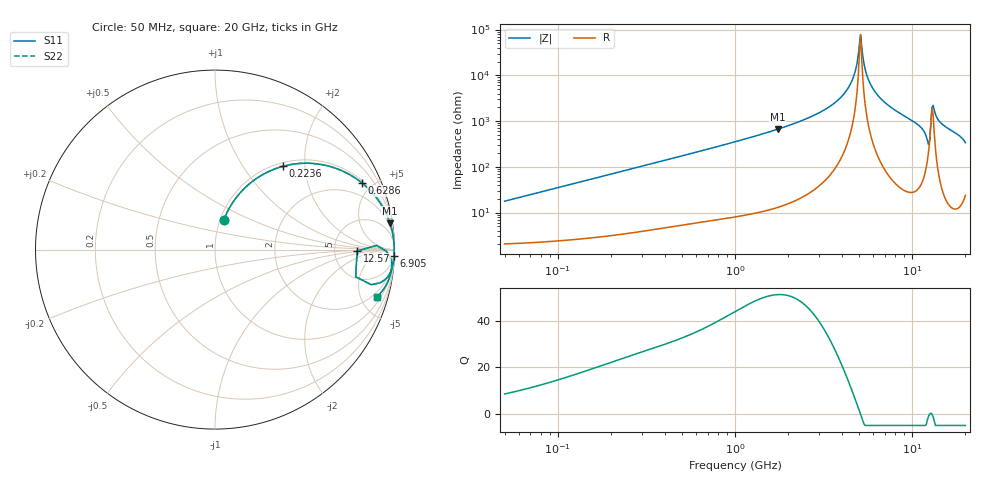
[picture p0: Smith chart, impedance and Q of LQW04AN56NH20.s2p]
!Murata Part Number: LQW04AN56NH20
!These Parameters are Measured in Series Mode Connection
!  o--[Z]--o
!Port1  Port2
!  o-------o
!Freq. Start=50[MHz] Stop=20[GHz], 401[Steps]
# Hz S RI R 50
!Freq.(Hz) S11(Real) S11(Imag) S21(Real) S21(Imag) S12(Real) S12(Imag) S22(Real) S22(Imag)
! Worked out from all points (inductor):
!   401 points, 50 MHz to 20 GHz, reference 50 ohm
!   read as one part in series: L = 55.8 nH near 51.52 MHz
!   highest Q = 51.3 at 1.741 GHz (marker M1), where L = 60.6 nH
!   self-resonance near 5.041 GHz
!   S11 on the Smith chart (normalised r, x): 50 MHz: 1.04, +0.35; 223.6 MHz: 1.07, +1.55; 628.6 MHz: 1.12, +4.35; 6.905 GHz: 3, -54; 12.57 GHz: 8.60, -0.37; 20 GHz: 1.48, -6.73
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5e7  0.0484 0.1639  0.9516 -0.1639  0.9516 -0.1639  0.0484 0.1639
1.364002e8  0.1976 0.3712  0.8024 -0.3712  0.8024 -0.3712  0.1976 0.3712
2.236068e8  0.3804 0.4646  0.6196 -0.4646  0.6196 -0.4646  0.3804 0.4646
3.721004e8  0.6188 0.4688  0.3812 -0.4688  0.3812 -0.4688  0.6188 0.4688
6.285508e8  0.8185 0.3717  0.1815 -0.3717  0.1815 -0.3717  0.8185 0.3717
1e9  0.9203 0.2597  0.0797 -0.2597  0.0797 -0.2597  0.9203 0.2597
1.740566e9  0.975 0.1466  0.025 -0.1466  0.025 -0.1466  0.975 0.1466
2.728004e9  0.9922 0.0774  0.00783 -0.0774  0.00783 -0.0774  0.9922 0.0774
3.572216e9  0.9967 0.0427  0.00329 -0.0427  0.00329 -0.0427  0.9967 0.0427
4.275624e9  0.9982 0.0211  0.00178 -0.0211  0.00178 -0.0211  0.9982 0.0211
4.677679e9  0.9986 0.0104  0.0014 -0.0104  0.0014 -0.0104  0.9986 0.0104
4.966507e9  0.9987 0.00337  0.00128 -0.00337  0.00128 -0.00337  0.9987 0.00337
5.117541e9  0.9987 -0.000168  0.00127 0.000168  0.00127 0.000168  0.9987 -0.000168
5.769027e9  0.9985 -0.0145  0.00146 0.0145  0.00146 0.0145  0.9985 -0.0145
6.905011e9  0.9973 -0.0369  0.00267 0.0369  0.00267 0.0369  0.9973 -0.0369
7.442007e9  0.9964 -0.0469  0.00357 0.0469  0.00357 0.0469  0.9964 -0.0469
1.082228e10  0.981 -0.1182  0.019 0.1182  0.019 0.1182  0.981 -0.1182
1.220001e10  0.87 -0.1956  0.13 0.1956  0.13 0.1956  0.87 -0.1956
1.257102e10  0.792 -0.00804  0.208 0.00804  0.208 0.00804  0.792 -0.00804
1.334722e10  0.9795 -0.0532  0.0205 0.0532  0.0205 0.0532  0.9795 -0.0532
1.460232e10  0.9831 -0.1096  0.0169 0.1096  0.0169 0.1096  0.9831 -0.1096
2e10  0.9036 -0.2618  0.0964 0.2618  0.0964 0.2618  0.9036 -0.2618
